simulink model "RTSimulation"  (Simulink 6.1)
settings: Solver=FixedStepDiscrete  StartTime=0.0  StopTime=inf  RelTol=1e-3
PreLoadFcn:
  | initialize
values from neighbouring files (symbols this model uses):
  actParams = [	bulkModulus   * pressCanon    [Copy of initialize.m]    (also in initialize.m = [bulkModulus	* pressCanon,)
  aLpf = [1]    [randth.m]
  bLpf = [1]    [randth.m]
  displFreq = inf    [initialize.m]
  flowCanon = 1.666667e+04    (= 16666.67)    [Copy of initialize.m]    (also in initialize.m)
  forceCanon = 1    [Copy of initialize.m]    (also in initialize.m)
  forceFreq = inf    [initialize.m]
  friction = 5			 				* 0.155000	 				* 0.00444822 				* area1    (= 2.71252900422)    [initialize.m]
  fsamp = 1 / samplePeriod    (= 1024)    [Copy of initialize.m]    (also in initialize.m; rampth.m = 1 / deltaT; randth.m = 1 / deltaT; rspect.m = 1.0 / tsamp)
  gasConstant = 1.8    [Copy of initialize.m]    (also in initialize.m)
  lengthCanon = 1    [Copy of initialize.m]    (also in initialize.m)
  massCanon = 1e-06    [Copy of initialize.m]    (also in initialize.m)
  maxDispl = ( (stroke2 + endLength2) * lengthCanon)'    [Copy of initialize.m]    (also in initialize.m = 576.2)
  maxOilVolume = volume * (1 - (precharge/supplyPress)^(1/gasConstant))    (= 211.391477114)    [Copy of initialize.m]    (also in initialize.m)
  maxVeloc = ( (maxFlow' * flowCanon ./ (area1 * areaCanon)) / velocCanon)'    [Copy of initialize.m]    (also in initialize.m = (maxFlow * flowCanon / (area1 * areaCanon)) / velocCanon; rampth.m = 2 * maxDispl / (nVeloc * deltaT))
  minDispl = (-(stroke1 + endLength1) * lengthCanon)'    [Copy of initialize.m]    (also in initialize.m = -576.2)
  minVeloc = (-(maxFlow' * flowCanon ./ (area2 * areaCanon)) / velocCanon)'    [Copy of initialize.m]    (also in initialize.m = -(maxFlow * flowCanon / (area2 * areaCanon)) / velocCanon)
  nAct = 5    [Copy of initialize.m]    (also in initialize.m = 1)
  nAdcU = 6    [Copy of initialize.m]    (also in initialize.m = 5)
  nDout = 4    [Copy of initialize.m]    (also in initialize.m)
  nDucU = 2    [Copy of initialize.m]    (also in initialize.m)
  nEncU = 3    [Copy of initialize.m]    (also in initialize.m)
  node = completenodestruct(node)    [Copy of initialize.m]    (also in initialize.m)
  precharge = 3000		 				* 6.894757e-03    (= 20.684271)    [Copy of initialize.m]    (also in initialize.m)
  pumpFlow = 1e20    (= 1e+20)    [Copy of initialize.m]    (also in initialize.m)
  returnPress = 3			 				* 0.1    (= 0.3)    [Copy of initialize.m]    (also in initialize.m)
  samplePeriod = controlPeriod/upsampleFactor    (= 0.0009765625)    [Copy of initialize.m]    (also in initialize.m; viewer.m = eval(getHeaderValue(header, 'DELTA_T')))
  springCanon = 1    [Copy of initialize.m]    (also in initialize.m)
  supplyPress = 280		 				* 0.1    (= 28)    [Copy of initialize.m]    (also in initialize.m)
  velocCanon = 1    [Copy of initialize.m]    (also in initialize.m)
  volume = 15.15		 				+ (  45		 				    * 2		 				   + 30		 				    * 6 )	 				* 5    (= 1365.15)    [Copy of initialize.m]    (also in initialize.m; quake.m = volume / 231.0)
  volumeCanon = 1e+06    (= 1000000)    [Copy of initialize.m]    (also in initialize.m)
  yieldDispl = 1.0    (= 1)    [initialize.m]
undefined symbols (not defined in the file or in its folder): DiscIntNeverNeededParam, dpforceFreq, mass, spring, staticForce
libraries: xpclib x6, simulink x1
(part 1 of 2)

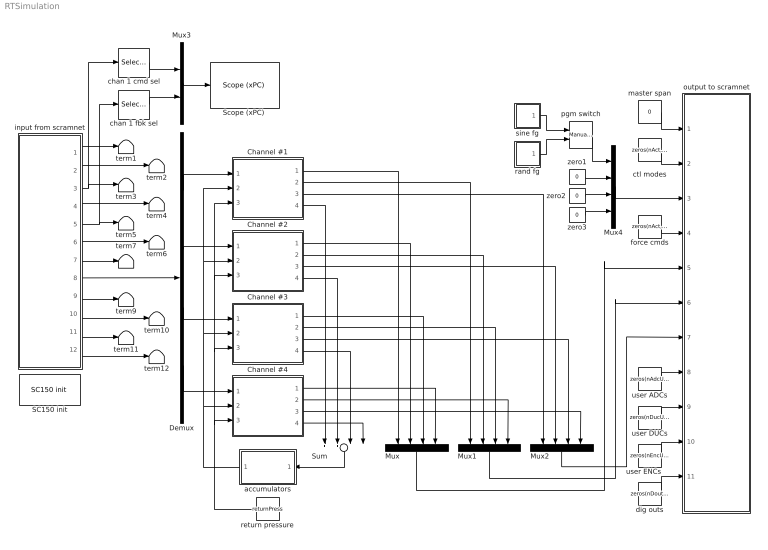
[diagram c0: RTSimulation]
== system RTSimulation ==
  Channel #1 : Subsystem  mask{id=1}
      mask prompts: id "Channel ID"
  Channel #2 : Subsystem  mask{id=2}
      mask prompts: id "Channel ID"
  Channel #3 : Subsystem  mask{id=3}
      mask prompts: id "Channel ID"
  Channel #4 : Subsystem  mask{id=4}
      mask prompts: id "Channel ID"
  Demux : Demux  Outputs=nAct
  Mux : Mux  Orientation=down  Inputs=nAct
  Mux1 : Mux  Orientation=down  Inputs=nAct
  Mux2 : Mux  Orientation=down  Inputs=nAct
  Mux3 : Mux  Inputs=2
  Mux4 : Mux  Inputs=nAct
  SC150 init : xpclib/Shared Memory/Systran/SC150 init   node=node  pci=-1
  "Scope (xPC) " : xpclib/Misc./Scope (xPC)   scopeno=2  scopetype=Target  autostart=on  viewmode=Graphical redraw  formatstr='%15.6f'  grid=on  ylimits=[0,0]  nosamples=1024  noprepostsamples=0  interleave=1  triggermode=FreeRun  triggersignal=1  triggerlevel=0.0  triggerslope=Either  triggerscope=1  triggersample=0  filename=data.dat  mode=Lazy  writesize=512  autorestart=off
  Sum : Sum  Orientation=down  Inputs=++++
  accumulators : Subsystem  Orientation=left
  chan 1 cmd sel : Selector
  chan 1 fbk sel : Selector
  ctl modes : Constant  Value=zeros(nAct, 1)
  dig outs : Constant  Value=zeros(nDout, 1)  OutDataTypeMode=uint32
  force cmds : Constant  Value=zeros(nAct, 1)
  input from scramnet : Subsystem
  master span : Constant  Value=0
  output to scramnet : Subsystem
  pgm switch : simulink/Signal Routing/Manual Switch  sw=1  action=0
  rand fg : Subsystem  mask(Sine Function Generator){ampl=1, bw=10, spanInterval=1, samplePeriod=samplePeriod}
      mask prompts: ampl "RMS amplitude"; bw "Bandwidth (Hz)"; spanInterval "Span interval (sec)"; samplePeriod "Sample period (sec)"
      mask init:
      | gain = ampl*sqrt(3)*sqrt(1/(2*samplePeriod*bw));
  return pressure : Constant  Orientation=left  Value=returnPress
  sine fg : Subsystem  mask(Sine Function Generator){ampl=1, freq=1, spanInterval=1, samplePeriod=samplePeriod}
      mask prompts: ampl "Amplitude"; freq "Frequency (Hz)"; spanInterval "Span interval (sec)"; samplePeriod "Sample period (sec)"
  term{1..7,9..12} (11 alike) : Terminator
  user ADCs : Constant  Value=zeros(nAdcU, 1)
  user DUCs : Constant  Value=zeros(nDucU, 1)
  user ENCs : Constant  Value=zeros(nEncU, 1)
  zero1 : Constant  Value=0
  zero2 : Constant  Value=0
  zero3 : Constant  Value=0
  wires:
  input from scramnet/6(force fbks) -> term6/1
  input from scramnet/10(user ducs) -> term10/1
  input from scramnet/12(dig inps) -> term12/1
  input from scramnet/4(force cmds) -> term4/1
  input from scramnet/5(displ fbks) -> term5/1, chan 1 fbk sel/1
  input from scramnet/7(dpforce fbks) -> term7/1
  input from scramnet/9(user adcs) -> term9/1
  input from scramnet/11(user encs) -> term11/1
  input from scramnet/1(master span) -> term1/1
  input from scramnet/2(ctl modes) -> term2/1
  input from scramnet/3(displ cmds) -> term3/1, chan 1 cmd sel/1
  master span/1 -> output to scramnet/1(master span)
  ctl modes/1 -> output to scramnet/2(ctl modes)
  force cmds/1 -> output to scramnet/4(force cmds)
  user ADCs/1 -> output to scramnet/8(user adcs)
  user DUCs/1 -> output to scramnet/9(user ducs)
  user ENCs/1 -> output to scramnet/10(user encs)
  dig outs/1 -> output to scramnet/11(dig outs)
  Channel #1/4(flow) -> Sum/1
  Channel #2/4(flow) -> Sum/2
  Channel #3/4(flow) -> Sum/3
  Sum/1 -> accumulators/1(flow)
  Channel #4/4(flow) -> Sum/4
  Channel #1/1(displ) -> Mux/1
  Channel #2/1(displ) -> Mux/2
  Channel #3/1(displ) -> Mux/3
  Channel #4/1(displ) -> Mux/4
  Channel #1/2(force) -> Mux1/1
  Channel #2/2(force) -> Mux1/2
  Channel #3/2(force) -> Mux1/3
  Channel #4/2(force) -> Mux1/4
  Channel #1/3(dpforce) -> Mux2/1
  Channel #2/3(dpforce) -> Mux2/2
  Channel #3/3(dpforce) -> Mux2/3
  Channel #4/3(dpforce) -> Mux2/4
  Mux/1 -> output to scramnet/5(displ fbks)
  Mux1/1 -> output to scramnet/6(force fbks)
  Mux2/1 -> output to scramnet/7(dpforce fbks)
  Demux/1 -> Channel #1/1(valve cmd)
  Demux/2 -> Channel #2/1(valve cmd)
  Demux/3 -> Channel #3/1(valve cmd)
  Demux/4 -> Channel #4/1(valve cmd)
  accumulators/1(press) -> Channel #3/2(spl press), Channel #2/2(spl press), Channel #1/2(spl press), Channel #4/2(spl press)
  return pressure/1 -> Channel #3/3(rtn press), Channel #2/3(rtn press), Channel #1/3(rtn press), Channel #4/3(rtn press)
  input from scramnet/8(valve cmds) -> Demux/1
  sine fg/1(out) -> pgm switch/1
  rand fg/1(out) -> pgm switch/2
  chan 1 cmd sel/1 -> Mux3/1
  chan 1 fbk sel/1 -> Mux3/2
  Mux3/1 -> "Scope (xPC) "/1
  zero1/1 -> Mux4/2
  zero2/1 -> Mux4/3
  zero3/1 -> Mux4/4
  Mux4/1 -> output to scramnet/3(displ cmds)
  pgm switch/1 -> Mux4/1

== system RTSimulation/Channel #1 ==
  valve cmd : Inport  Port=1  LatchInput=off
  spl press : Inport  Port=2  LatchInput=off
  rtn press : Inport  Port=3  LatchInput=off
  actuator/valve  model : Subsystem
  displ cond filter : Subsystem  mask{freq3dB=displFreq(id), fsamp=fsamp}
      mask prompts: freq3dB "3 dB cutoff frequency (inf, 500, 300, 100, 50 Hz)"; fsamp "Sampling frequency (Hz)"
      mask init:
      | if isempty(freq3dB)
      | 	freq3dB = fsamp;
      | elseif freq3dB == 500
      | 	freq3dB = 485;
      | elseif freq3dB == 300
      | 	freq3dB = 204.9;
      | elseif freq3dB == 100
      | 	freq3dB = 56.5;
      | elseif freq3dB == 50
      | 	freq3dB = 27.8;
      | else
      | 	freq3dB = fsamp;
      | end
      | if freq3dB > fsamp/2
      | 	a = [1];
      | 	b = [1];
      | else
      | 	[b, a] = ellip(4, 0.001, 60.0, 2*freq3dB/fsamp);
      | end
  dpforce cond filter : Subsystem  mask{freq3dB=dpforceFreq(id), fsamp=fsamp}
      mask prompts: freq3dB "3 dB cutoff frequency (inf, 500, 300, 100, 50 Hz)"; fsamp "Sampling frequency (Hz)"
      mask init:
      | if isempty(freq3dB)
      | 	freq3dB = fsamp;
      | elseif freq3dB == 500
      | 	freq3dB = 485;
      | elseif freq3dB == 300
      | 	freq3dB = 204.9;
      | elseif freq3dB == 100
      | 	freq3dB = 56.5;
      | elseif freq3dB == 50
      | 	freq3dB = 27.8;
      | else
      | 	freq3dB = fsamp;
      | end
      | if freq3dB > fsamp/2
      | 	a = [1];
      | 	b = [1];
      | else
      | 	[b, a] = ellip(4, 0.001, 60.0, 2*freq3dB/fsamp);
      | end
  force cond filter : Subsystem  mask{freq3dB=forceFreq((id)), fsamp=fsamp}
      mask prompts: freq3dB "3 dB cutoff frequency (inf, 500, 300, 100, 50 Hz)"; fsamp "Sampling frequency (Hz)"
      mask init:
      | if isempty(freq3dB)
      | 	freq3dB = fsamp;
      | elseif freq3dB == 500
      | 	freq3dB = 485;
      | elseif freq3dB == 300
      | 	freq3dB = 204.9;
      | elseif freq3dB == 100
      | 	freq3dB = 56.5;
      | elseif freq3dB == 50
      | 	freq3dB = 27.8;
      | else
      | 	freq3dB = fsamp;
      | end
      | if freq3dB > fsamp/2
      | 	a = [1];
      | 	b = [1];
      | else
      | 	[b, a] = ellip(4, 0.001, 60.0, 2*freq3dB/fsamp);
      | end
  payload : Subsystem
  displ : Outport
  force : Outport  Port=2
  dpforce : Outport  Port=3
  flow : Outport  Port=4
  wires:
  dpforce cond filter/1(out) -> dpforce/1
  force cond filter/1(out) -> force/1
  displ cond filter/1(out) -> displ/1
  actuator/valve  model/1(force) -> payload/1(force), dpforce cond filter/1(inp), force cond filter/1(inp)
  actuator/valve  model/2(flow) -> flow/1
  spl press/1 -> actuator/valve  model/4(spl press)
  rtn press/1 -> actuator/valve  model/5(rtn press)
  valve cmd/1 -> actuator/valve  model/1(cmd)
  payload/1(displ) -> displ cond filter/1(inp), actuator/valve  model/2(displ)
  payload/2(veloc) -> actuator/valve  model/3(veloc)

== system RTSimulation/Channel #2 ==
  valve cmd : Inport  Port=1  LatchInput=off
  spl press : Inport  Port=2  LatchInput=off
  rtn press : Inport  Port=3  LatchInput=off
  actuator/valve  model : Subsystem
  displ cond filter : Subsystem  mask{freq3dB=displFreq(id), fsamp=fsamp}
      mask prompts: freq3dB "3 dB cutoff frequency (inf, 500, 300, 100, 50 Hz)"; fsamp "Sampling frequency (Hz)"
      mask init:
      | if isempty(freq3dB)
      | 	freq3dB = fsamp;
      | elseif freq3dB == 500
      | 	freq3dB = 485;
      | elseif freq3dB == 300
      | 	freq3dB = 204.9;
      | elseif freq3dB == 100
      | 	freq3dB = 56.5;
      | elseif freq3dB == 50
      | 	freq3dB = 27.8;
      | else
      | 	freq3dB = fsamp;
      | end
      | if freq3dB > fsamp/2
      | 	a = [1];
      | 	b = [1];
      | else
      | 	[b, a] = ellip(4, 0.001, 60.0, 2*freq3dB/fsamp);
      | end
  dpforce cond filter : Subsystem  mask{freq3dB=dpforceFreq(id), fsamp=fsamp}
      mask prompts: freq3dB "3 dB cutoff frequency (inf, 500, 300, 100, 50 Hz)"; fsamp "Sampling frequency (Hz)"
      mask init:
      | if isempty(freq3dB)
      | 	freq3dB = fsamp;
      | elseif freq3dB == 500
      | 	freq3dB = 485;
      | elseif freq3dB == 300
      | 	freq3dB = 204.9;
      | elseif freq3dB == 100
      | 	freq3dB = 56.5;
      | elseif freq3dB == 50
      | 	freq3dB = 27.8;
      | else
      | 	freq3dB = fsamp;
      | end
      | if freq3dB > fsamp/2
      | 	a = [1];
      | 	b = [1];
      | else
      | 	[b, a] = ellip(4, 0.001, 60.0, 2*freq3dB/fsamp);
      | end
  force cond filter : Subsystem  mask{freq3dB=forceFreq((id)), fsamp=fsamp}
      mask prompts: freq3dB "3 dB cutoff frequency (inf, 500, 300, 100, 50 Hz)"; fsamp "Sampling frequency (Hz)"
      mask init:
      | if isempty(freq3dB)
      | 	freq3dB = fsamp;
      | elseif freq3dB == 500
      | 	freq3dB = 485;
      | elseif freq3dB == 300
      | 	freq3dB = 204.9;
      | elseif freq3dB == 100
      | 	freq3dB = 56.5;
      | elseif freq3dB == 50
      | 	freq3dB = 27.8;
      | else
      | 	freq3dB = fsamp;
      | end
      | if freq3dB > fsamp/2
      | 	a = [1];
      | 	b = [1];
      | else
      | 	[b, a] = ellip(4, 0.001, 60.0, 2*freq3dB/fsamp);
      | end
  payload : Subsystem
  displ : Outport
  force : Outport  Port=2
  dpforce : Outport  Port=3
  flow : Outport  Port=4
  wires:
  payload/2(veloc) -> actuator/valve  model/3(veloc)
  payload/1(displ) -> actuator/valve  model/2(displ), displ cond filter/1(inp)
  valve cmd/1 -> actuator/valve  model/1(cmd)
  rtn press/1 -> actuator/valve  model/5(rtn press)
  spl press/1 -> actuator/valve  model/4(spl press)
  actuator/valve  model/2(flow) -> flow/1
  actuator/valve  model/1(force) -> force cond filter/1(inp), dpforce cond filter/1(inp), payload/1(force)
  displ cond filter/1(out) -> displ/1
  force cond filter/1(out) -> force/1
  dpforce cond filter/1(out) -> dpforce/1

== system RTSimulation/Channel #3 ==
  valve cmd : Inport  Port=1  LatchInput=off
  spl press : Inport  Port=2  LatchInput=off
  rtn press : Inport  Port=3  LatchInput=off
  actuator/valve  model : Subsystem
  displ cond filter : Subsystem  mask{freq3dB=displFreq(id), fsamp=fsamp}
      mask prompts: freq3dB "3 dB cutoff frequency (inf, 500, 300, 100, 50 Hz)"; fsamp "Sampling frequency (Hz)"
      mask init:
      | if isempty(freq3dB)
      | 	freq3dB = fsamp;
      | elseif freq3dB == 500
      | 	freq3dB = 485;
      | elseif freq3dB == 300
      | 	freq3dB = 204.9;
      | elseif freq3dB == 100
      | 	freq3dB = 56.5;
      | elseif freq3dB == 50
      | 	freq3dB = 27.8;
      | else
      | 	freq3dB = fsamp;
      | end
      | if freq3dB > fsamp/2
      | 	a = [1];
      | 	b = [1];
      | else
      | 	[b, a] = ellip(4, 0.001, 60.0, 2*freq3dB/fsamp);
      | end
  dpforce cond filter : Subsystem  mask{freq3dB=dpforceFreq(id), fsamp=fsamp}
      mask prompts: freq3dB "3 dB cutoff frequency (inf, 500, 300, 100, 50 Hz)"; fsamp "Sampling frequency (Hz)"
      mask init:
      | if isempty(freq3dB)
      | 	freq3dB = fsamp;
      | elseif freq3dB == 500
      | 	freq3dB = 485;
      | elseif freq3dB == 300
      | 	freq3dB = 204.9;
      | elseif freq3dB == 100
      | 	freq3dB = 56.5;
      | elseif freq3dB == 50
      | 	freq3dB = 27.8;
      | else
      | 	freq3dB = fsamp;
      | end
      | if freq3dB > fsamp/2
      | 	a = [1];
      | 	b = [1];
      | else
      | 	[b, a] = ellip(4, 0.001, 60.0, 2*freq3dB/fsamp);
      | end
  force cond filter : Subsystem  mask{freq3dB=forceFreq((id)), fsamp=fsamp}
      mask prompts: freq3dB "3 dB cutoff frequency (inf, 500, 300, 100, 50 Hz)"; fsamp "Sampling frequency (Hz)"
      mask init:
      | if isempty(freq3dB)
      | 	freq3dB = fsamp;
      | elseif freq3dB == 500
      | 	freq3dB = 485;
      | elseif freq3dB == 300
      | 	freq3dB = 204.9;
      | elseif freq3dB == 100
      | 	freq3dB = 56.5;
      | elseif freq3dB == 50
      | 	freq3dB = 27.8;
      | else
      | 	freq3dB = fsamp;
      | end
      | if freq3dB > fsamp/2
      | 	a = [1];
      | 	b = [1];
      | else
      | 	[b, a] = ellip(4, 0.001, 60.0, 2*freq3dB/fsamp);
      | end
  payload : Subsystem
  displ : Outport
  force : Outport  Port=2
  dpforce : Outport  Port=3
  flow : Outport  Port=4
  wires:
  dpforce cond filter/1(out) -> dpforce/1
  force cond filter/1(out) -> force/1
  displ cond filter/1(out) -> displ/1
  actuator/valve  model/1(force) -> payload/1(force), dpforce cond filter/1(inp), force cond filter/1(inp)
  actuator/valve  model/2(flow) -> flow/1
  spl press/1 -> actuator/valve  model/4(spl press)
  rtn press/1 -> actuator/valve  model/5(rtn press)
  valve cmd/1 -> actuator/valve  model/1(cmd)
  payload/1(displ) -> displ cond filter/1(inp), actuator/valve  model/2(displ)
  payload/2(veloc) -> actuator/valve  model/3(veloc)

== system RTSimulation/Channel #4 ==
  valve cmd : Inport  Port=1  LatchInput=off
  spl press : Inport  Port=2  LatchInput=off
  rtn press : Inport  Port=3  LatchInput=off
  actuator/valve  model : Subsystem
  displ cond filter : Subsystem  mask{freq3dB=displFreq(id), fsamp=fsamp}
      mask prompts: freq3dB "3 dB cutoff frequency (inf, 500, 300, 100, 50 Hz)"; fsamp "Sampling frequency (Hz)"
      mask init:
      | if isempty(freq3dB)
      | 	freq3dB = fsamp;
      | elseif freq3dB == 500
      | 	freq3dB = 485;
      | elseif freq3dB == 300
      | 	freq3dB = 204.9;
      | elseif freq3dB == 100
      | 	freq3dB = 56.5;
      | elseif freq3dB == 50
      | 	freq3dB = 27.8;
      | else
      | 	freq3dB = fsamp;
      | end
      | if freq3dB > fsamp/2
      | 	a = [1];
      | 	b = [1];
      | else
      | 	[b, a] = ellip(4, 0.001, 60.0, 2*freq3dB/fsamp);
      | end
  dpforce cond filter : Subsystem  mask{freq3dB=dpforceFreq(id), fsamp=fsamp}
      mask prompts: freq3dB "3 dB cutoff frequency (inf, 500, 300, 100, 50 Hz)"; fsamp "Sampling frequency (Hz)"
      mask init:
      | if isempty(freq3dB)
      | 	freq3dB = fsamp;
      | elseif freq3dB == 500
      | 	freq3dB = 485;
      | elseif freq3dB == 300
      | 	freq3dB = 204.9;
      | elseif freq3dB == 100
      | 	freq3dB = 56.5;
      | elseif freq3dB == 50
      | 	freq3dB = 27.8;
      | else
      | 	freq3dB = fsamp;
      | end
      | if freq3dB > fsamp/2
      | 	a = [1];
      | 	b = [1];
      | else
      | 	[b, a] = ellip(4, 0.001, 60.0, 2*freq3dB/fsamp);
      | end
  force cond filter : Subsystem  mask{freq3dB=forceFreq((id)), fsamp=fsamp}
      mask prompts: freq3dB "3 dB cutoff frequency (inf, 500, 300, 100, 50 Hz)"; fsamp "Sampling frequency (Hz)"
      mask init:
      | if isempty(freq3dB)
      | 	freq3dB = fsamp;
      | elseif freq3dB == 500
      | 	freq3dB = 485;
      | elseif freq3dB == 300
      | 	freq3dB = 204.9;
      | elseif freq3dB == 100
      | 	freq3dB = 56.5;
      | elseif freq3dB == 50
      | 	freq3dB = 27.8;
      | else
      | 	freq3dB = fsamp;
      | end
      | if freq3dB > fsamp/2
      | 	a = [1];
      | 	b = [1];
      | else
      | 	[b, a] = ellip(4, 0.001, 60.0, 2*freq3dB/fsamp);
      | end
  payload : Subsystem
  displ : Outport
  force : Outport  Port=2
  dpforce : Outport  Port=3
  flow : Outport  Port=4
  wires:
  payload/2(veloc) -> actuator/valve  model/3(veloc)
  payload/1(displ) -> actuator/valve  model/2(displ), displ cond filter/1(inp)
  valve cmd/1 -> actuator/valve  model/1(cmd)
  rtn press/1 -> actuator/valve  model/5(rtn press)
  spl press/1 -> actuator/valve  model/4(spl press)
  actuator/valve  model/2(flow) -> flow/1
  actuator/valve  model/1(force) -> force cond filter/1(inp), dpforce cond filter/1(inp), payload/1(force)
  displ cond filter/1(out) -> displ/1
  force cond filter/1(out) -> force/1
  dpforce cond filter/1(out) -> dpforce/1

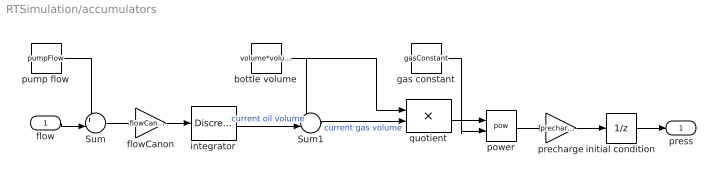
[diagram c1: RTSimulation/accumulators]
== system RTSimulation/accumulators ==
  flow : Inport  Port=1  LatchInput=off
  Sum : Sum  Inputs=+-|
  Sum1 : Sum  Inputs=+-|
  bottle volume : Constant  Value=volume*volumeCanon
  flowCanon : Gain  Gain=flowCanon
  gas constant : Constant  Value=gasConstant
  initial condition : UnitDelay  X0=supplyPress  SampleTime=-1
  integrator : DiscreteIntegrator  InitialCondition=maxOilVolume*volumeCanon  SampleTime=-1  LimitOutput=on  UpperSaturationLimit=maxOilVolume*volumeCanon  LowerSaturationLimit=0  ICPrevOutput=DiscIntNeverNeededParam  ICPrevScaledInput=DiscIntNeverNeededParam
  power : Math  Operator=pow
  precharge : Gain  Gain=precharge
  pump flow : Constant  Value=pumpFlow
  quotient : Product  Inputs=*/
  press : Outport
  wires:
  pump flow/1 -> Sum/1
  Sum/1 -> flowCanon/1
  bottle volume/1 -> Sum1/1, quotient/1
  gas constant/1 -> power/2
  power/1 -> precharge/1
  precharge/1 -> initial condition/1
  Sum1/1 -> quotient/2  "current gas volume"
  quotient/1 -> power/1
  integrator/1 -> Sum1/2  "current oil volume"
  flow/1 -> Sum/2
  flowCanon/1 -> integrator/1
  initial condition/1 -> press/1

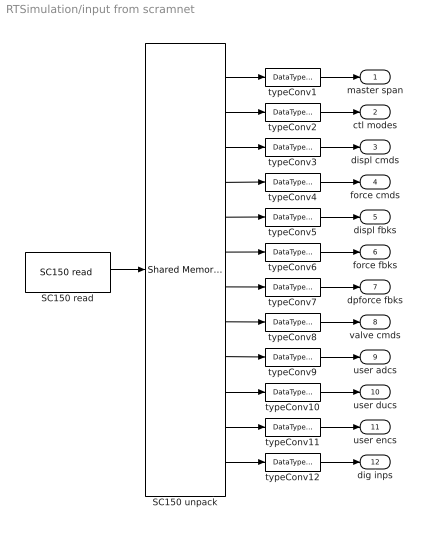
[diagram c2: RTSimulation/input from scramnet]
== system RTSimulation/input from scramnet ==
  SC150 read : xpclib/Shared Memory/Systran/SC150 read   partition=node.Partitions(12:23)  ts=samplePeriod  pci=-1
  SC150 unpack : xpclib/Shared Memory/Shared Memory Unpack   partition=node.Partitions(12:23)
  typeConv{1,3..11} (10 alike) : DataTypeConversion  OutDataTypeMode=double
  typeConv12 : DataTypeConversion  OutDataTypeMode=uint32
  typeConv2 : DataTypeConversion  OutDataTypeMode=uint32
  master span : Outport
  ctl modes : Outport  Port=2
  displ cmds : Outport  Port=3
  force cmds : Outport  Port=4
  displ fbks : Outport  Port=5
  force fbks : Outport  Port=6
  dpforce fbks : Outport  Port=7
  valve cmds : Outport  Port=8
  user adcs : Outport  Port=9
  user ducs : Outport  Port=10
  user encs : Outport  Port=11
  dig inps : Outport  Port=12
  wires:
  typeConv11/1 -> user encs/1
  typeConv10/1 -> user ducs/1
  typeConv12/1 -> dig inps/1
  typeConv9/1 -> user adcs/1
  typeConv8/1 -> valve cmds/1
  typeConv7/1 -> dpforce fbks/1
  typeConv6/1 -> force fbks/1
  typeConv5/1 -> displ fbks/1
  typeConv4/1 -> force cmds/1
  typeConv3/1 -> displ cmds/1
  typeConv1/1 -> master span/1
  SC150 read/1 -> SC150 unpack/1
  typeConv2/1 -> ctl modes/1
  SC150 unpack/1 -> typeConv1/1
  SC150 unpack/2 -> typeConv2/1
  SC150 unpack/3 -> typeConv3/1
  SC150 unpack/4 -> typeConv4/1
  SC150 unpack/5 -> typeConv5/1
  SC150 unpack/6 -> typeConv6/1
  SC150 unpack/7 -> typeConv7/1
  SC150 unpack/8 -> typeConv8/1
  SC150 unpack/9 -> typeConv9/1
  SC150 unpack/10 -> typeConv10/1
  SC150 unpack/11 -> typeConv11/1
  SC150 unpack/12 -> typeConv12/1

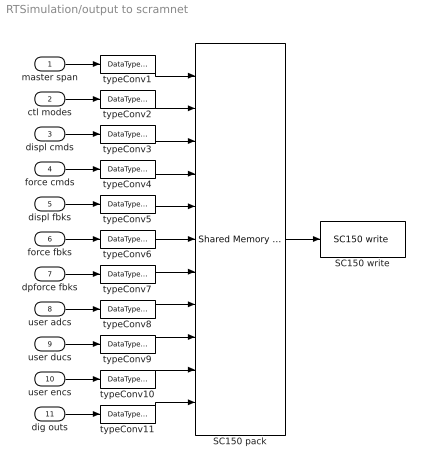
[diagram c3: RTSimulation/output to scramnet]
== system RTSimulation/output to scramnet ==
  master span : Inport  Port=1  LatchInput=off
  ctl modes : Inport  Port=2  LatchInput=off
  displ cmds : Inport  Port=3  LatchInput=off
  force cmds : Inport  Port=4  LatchInput=off
  displ fbks : Inport  Port=5  LatchInput=off
  force fbks : Inport  Port=6  LatchInput=off
  dpforce fbks : Inport  Port=7  LatchInput=off
  user adcs : Inport  Port=8  LatchInput=off
  user ducs : Inport  Port=9  LatchInput=off
  user encs : Inport  Port=10  LatchInput=off
  dig outs : Inport  Port=11  LatchInput=off
  SC150 pack : xpclib/Shared Memory/Shared Memory Pack   partition=node.Partitions(1:11)
  SC150 write : xpclib/Shared Memory/Systran/SC150 write   partition=node.Partitions(1:11)  ts=samplePeriod  pci=-1
  typeConv{1,3..10} (9 alike) : DataTypeConversion  OutDataTypeMode=single
  typeConv11 : DataTypeConversion  OutDataTypeMode=uint32
  typeConv2 : DataTypeConversion  OutDataTypeMode=uint32
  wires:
  typeConv11/1 -> SC150 pack/11
  typeConv10/1 -> SC150 pack/10
  typeConv9/1 -> SC150 pack/9
  typeConv8/1 -> SC150 pack/8
  typeConv7/1 -> SC150 pack/7
  typeConv6/1 -> SC150 pack/6
  typeConv5/1 -> SC150 pack/5
  dig outs/1 -> typeConv11/1
  user encs/1 -> typeConv10/1
  user ducs/1 -> typeConv9/1
  user adcs/1 -> typeConv8/1
  dpforce fbks/1 -> typeConv7/1
  force fbks/1 -> typeConv6/1
  displ fbks/1 -> typeConv5/1
  force cmds/1 -> typeConv4/1
  master span/1 -> typeConv1/1
  SC150 pack/1 -> SC150 write/1
  displ cmds/1 -> typeConv3/1
  ctl modes/1 -> typeConv2/1
  typeConv1/1 -> SC150 pack/1
  typeConv2/1 -> SC150 pack/2
  typeConv3/1 -> SC150 pack/3
  typeConv4/1 -> SC150 pack/4

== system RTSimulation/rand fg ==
  Product : Product
  integrator : DiscreteIntegrator  SampleTime=-1  LimitOutput=on  UpperSaturationLimit=1  LowerSaturationLimit=0  ICPrevOutput=DiscIntNeverNeededParam  ICPrevScaledInput=DiscIntNeverNeededParam
  lowpass : Subsystem  mask{freq=bw, k=gain, samplePeriod=samplePeriod}
      mask prompts: freq "Cutoff frequency (Hz)"; k "Gain"; samplePeriod "Sample period (sec)"
      mask init:
      | damp = sqrt(2);
      | b = [0 0 (2*pi*freq)^2];
      | a = [1 2*(2*pi*freq)*damp (2*pi*freq)^2];
      | [bLpf aLpf] = bilinear(b, a, 1/samplePeriod);
  span rate : Constant  Value=1/spanInterval
  uniform rand : UniformRandomNumber  SampleTime=samplePeriod
  out : Outport
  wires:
  integrator/1 -> Product/2
  span rate/1 -> integrator/1
  Product/1 -> out/1
  uniform rand/1 -> lowpass/1(inp)
  lowpass/1(out) -> Product/1

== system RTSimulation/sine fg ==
  Product : Product
  integrator : DiscreteIntegrator  SampleTime=-1  LimitOutput=on  UpperSaturationLimit=1  LowerSaturationLimit=0  ICPrevOutput=DiscIntNeverNeededParam  ICPrevScaledInput=DiscIntNeverNeededParam
  sine : Sin  Amplitude=ampl  Frequency=2 * pi * freq  SampleTime=samplePeriod
  span rate : Constant  Value=1/spanInterval
  out : Outport
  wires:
  Product/1 -> out/1
  sine/1 -> Product/1
  span rate/1 -> integrator/1
  integrator/1 -> Product/2

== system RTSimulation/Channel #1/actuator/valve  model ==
  note: Parameter vector: 1: oil bulk modulus (force/displ^2) 2: servovalve delay (sec) 3: servovalve overlap 4: rated pressure (force/displ^2) 5: rated flow at rated pressure (displ^3/sec) 6: nominal flow at rated pressure (displ^3/sec) 7: actuator piston area 1 (displ^2) 8: actuator piston area 2 (displ^2) 9: actuator usable stroke 1 (displ) 10: actuator usable stroke 2 (displ) 11: actuator end cushion length 1 (displ) 12: actuator end cushion length 2 (displ) 13: actuator parasitic damping factor 14: cross-chamber leakage factor (flow/press) 15: ratio port openings according to area 16: sample period (sec) Conversion factors used for converting signals from external (user) to internal (canonical) units: 17: displacement 18: velocity 19: force 20: pressure 21: flow
  note: Auxiliary diagnostic output vector: 1: valve opening 2: C1 pressure 3: C2 pressure 4: delta pressure 5: force 6: velocity 7: C1 flow 8: C2 flow 9: total flow 10: kinematic flow 11: compressibility flow 12: leakage flow
  note: Note: "1" and "2" denote actuator cylinders on either side of the actuator piston. With positive valve drive, oil is ported into cylinder 1, resulting in positive displacement.
  cmd : Inport  Port=1  LatchInput=off
  displ : Inport  Port=2  LatchInput=off
  veloc : Inport  Port=3  LatchInput=off
  spl press : Inport  Port=4  LatchInput=off
  rtn press : Inport  Port=5  LatchInput=off
  abs : Abs
  actuator : S-Function  FunctionName=actuator  Parameters=actParams(:,id)
  total flow sel : Selector  Elements=9  InputPortWidth=12
  force : Outport
  flow : Outport  Port=2
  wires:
  abs/1 -> flow/1
  actuator/2 -> total flow sel/1
  total flow sel/1 -> abs/1
  spl press/1 -> actuator/4
  rtn press/1 -> actuator/5
  cmd/1 -> actuator/1
  actuator/1 -> force/1
  displ/1 -> actuator/2
  veloc/1 -> actuator/3

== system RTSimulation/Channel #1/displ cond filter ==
  inp : Inport  Port=1  LatchInput=off
  filter : DiscreteFilter  Numerator=b  Denominator=a  SampleTime=-1
  out : Outport
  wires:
  filter/1 -> out/1
  inp/1 -> filter/1

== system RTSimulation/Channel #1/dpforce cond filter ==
  inp : Inport  Port=1  LatchInput=off
  filter : DiscreteFilter  Numerator=b  Denominator=a  SampleTime=-1
  out : Outport
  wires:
  inp/1 -> filter/1
  filter/1 -> out/1

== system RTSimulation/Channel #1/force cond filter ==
  inp : Inport  Port=1  LatchInput=off
  filter : DiscreteFilter  Numerator=b  Denominator=a  SampleTime=-1
  out : Outport
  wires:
  filter/1 -> out/1
  inp/1 -> filter/1

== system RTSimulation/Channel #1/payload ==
  force : Inport  Port=1  LatchInput=off
  Sum : Sum  Inputs=+---
  displ gen : DiscreteIntegrator  IntegratorMethod=Integration: Backward Euler  SampleTime=-1  LimitOutput=on  UpperSaturationLimit=maxDispl(id)  LowerSaturationLimit=minDispl(id)  ShowSaturationPort=on  ICPrevOutput=DiscIntNeverNeededParam  ICPrevScaledInput=DiscIntNeverNeededParam
  div : Product  Inputs=*/
  friction : Subsystem  Orientation=left  mask{friction=friction(id)*forceCanon, yieldDispl=yieldDispl(id)*lengthCanon, hysteresis=0}
      mask prompts: friction "Sliding friction"; yieldDispl "Equiv. yield displacement (in)"; hysteresis "Hysteresis constant"
  mass : Constant  Value=mass(id)*massCanon
  spring : Gain  Orientation=left  Gain=spring(id)*springCanon
  static force : Constant  Value=staticForce(id)*forceCanon
  unit dly : UnitDelay  Orientation=left  SampleTime=-1
  veloc gen : Subsystem  mask{maxVeloc=maxVeloc(id)*velocCanon, minVeloc=minVeloc(id)*velocCanon, maxDispl=maxDispl(id), minDispl=minDispl(id)}
      mask prompts: maxVeloc "Max velocity"; minVeloc "Min velocity"; maxDispl "Max displacement"; minDispl "Min displacement"
  veloc units : Gain  Gain=1/velocCanon
  displ : Outport
  veloc : Outport  Port=2
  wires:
  spring/1 -> Sum/3  "spring force"
  mass/1 -> div/2
  force/1 -> Sum/1  "total force"
  static force/1 -> Sum/4  "static force"
  Sum/1 -> div/1  "inertial force"
  veloc units/1 -> veloc/1
  unit dly/1 -> spring/1
  friction/1(force) -> Sum/2  "friction force"
  displ gen/2 -> veloc gen/3(reset)
  displ gen/1 -> veloc gen/2(displ), unit dly/1, displ/1
  veloc gen/1(veloc) -> displ gen/1, veloc units/1, friction/1(veloc)
  div/1 -> veloc gen/1(accel)

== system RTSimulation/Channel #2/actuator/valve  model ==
  note: Note: "1" and "2" denote actuator cylinders on either side of the actuator piston. With positive valve drive, oil is ported into cylinder 1, resulting in positive displacement.
  note: Auxiliary diagnostic output vector: 1: valve opening 2: C1 pressure 3: C2 pressure 4: delta pressure 5: force 6: velocity 7: C1 flow 8: C2 flow 9: total flow 10: kinematic flow 11: compressibility flow 12: leakage flow
  note: Parameter vector: 1: oil bulk modulus (force/displ^2) 2: servovalve delay (sec) 3: servovalve overlap 4: rated pressure (force/displ^2) 5: rated flow at rated pressure (displ^3/sec) 6: nominal flow at rated pressure (displ^3/sec) 7: actuator piston area 1 (displ^2) 8: actuator piston area 2 (displ^2) 9: actuator usable stroke 1 (displ) 10: actuator usable stroke 2 (displ) 11: actuator end cushion length 1 (displ) 12: actuator end cushion length 2 (displ) 13: actuator parasitic damping factor 14: cross-chamber leakage factor (flow/press) 15: ratio port openings according to area 16: sample period (sec) Conversion factors used for converting signals from external (user) to internal (canonical) units: 17: displacement 18: velocity 19: force 20: pressure 21: flow
  cmd : Inport  Port=1  LatchInput=off
  displ : Inport  Port=2  LatchInput=off
  veloc : Inport  Port=3  LatchInput=off
  spl press : Inport  Port=4  LatchInput=off
  rtn press : Inport  Port=5  LatchInput=off
  abs : Abs
  actuator : S-Function  FunctionName=actuator  Parameters=actParams(:,id)
  total flow sel : Selector  Elements=9  InputPortWidth=12
  force : Outport
  flow : Outport  Port=2
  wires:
  veloc/1 -> actuator/3
  displ/1 -> actuator/2
  actuator/1 -> force/1
  cmd/1 -> actuator/1
  rtn press/1 -> actuator/5
  spl press/1 -> actuator/4
  total flow sel/1 -> abs/1
  actuator/2 -> total flow sel/1
  abs/1 -> flow/1

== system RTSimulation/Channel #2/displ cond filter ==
  inp : Inport  Port=1  LatchInput=off
  filter : DiscreteFilter  Numerator=b  Denominator=a  SampleTime=-1
  out : Outport
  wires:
  inp/1 -> filter/1
  filter/1 -> out/1

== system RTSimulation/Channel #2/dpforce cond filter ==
  inp : Inport  Port=1  LatchInput=off
  filter : DiscreteFilter  Numerator=b  Denominator=a  SampleTime=-1
  out : Outport
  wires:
  filter/1 -> out/1
  inp/1 -> filter/1

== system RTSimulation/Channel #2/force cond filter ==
  inp : Inport  Port=1  LatchInput=off
  filter : DiscreteFilter  Numerator=b  Denominator=a  SampleTime=-1
  out : Outport
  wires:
  inp/1 -> filter/1
  filter/1 -> out/1

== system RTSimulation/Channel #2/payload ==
  force : Inport  Port=1  LatchInput=off
  Sum : Sum  Inputs=+---
  displ gen : DiscreteIntegrator  IntegratorMethod=Integration: Backward Euler  SampleTime=-1  LimitOutput=on  UpperSaturationLimit=maxDispl(id)  LowerSaturationLimit=minDispl(id)  ShowSaturationPort=on  ICPrevOutput=DiscIntNeverNeededParam  ICPrevScaledInput=DiscIntNeverNeededParam
  div : Product  Inputs=*/
  friction : Subsystem  Orientation=left  mask{friction=friction(id)*forceCanon, yieldDispl=yieldDispl(id)*lengthCanon, hysteresis=0}
      mask prompts: friction "Sliding friction"; yieldDispl "Equiv. yield displacement (in)"; hysteresis "Hysteresis constant"
  mass : Constant  Value=mass(id)*massCanon
  spring : Gain  Orientation=left  Gain=spring(id)*springCanon
  static force : Constant  Value=staticForce(id)*forceCanon
  unit dly : UnitDelay  Orientation=left  SampleTime=-1
  veloc gen : Subsystem  mask{maxVeloc=maxVeloc(id)*velocCanon, minVeloc=minVeloc(id)*velocCanon, maxDispl=maxDispl(id), minDispl=minDispl(id)}
      mask prompts: maxVeloc "Max velocity"; minVeloc "Min velocity"; maxDispl "Max displacement"; minDispl "Min displacement"
  veloc units : Gain  Gain=1/velocCanon
  displ : Outport
  veloc : Outport  Port=2
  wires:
  div/1 -> veloc gen/1(accel)
  veloc gen/1(veloc) -> friction/1(veloc), veloc units/1, displ gen/1
  displ gen/1 -> displ/1, unit dly/1, veloc gen/2(displ)
  displ gen/2 -> veloc gen/3(reset)
  friction/1(force) -> Sum/2  "friction force"
  unit dly/1 -> spring/1
  veloc units/1 -> veloc/1
  Sum/1 -> div/1  "inertial force"
  static force/1 -> Sum/4  "static force"
  force/1 -> Sum/1  "total force"
  mass/1 -> div/2
  spring/1 -> Sum/3  "spring force"

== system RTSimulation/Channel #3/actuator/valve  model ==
  note: Parameter vector: 1: oil bulk modulus (force/displ^2) 2: servovalve delay (sec) 3: servovalve overlap 4: rated pressure (force/displ^2) 5: rated flow at rated pressure (displ^3/sec) 6: nominal flow at rated pressure (displ^3/sec) 7: actuator piston area 1 (displ^2) 8: actuator piston area 2 (displ^2) 9: actuator usable stroke 1 (displ) 10: actuator usable stroke 2 (displ) 11: actuator end cushion length 1 (displ) 12: actuator end cushion length 2 (displ) 13: actuator parasitic damping factor 14: cross-chamber leakage factor (flow/press) 15: ratio port openings according to area 16: sample period (sec) Conversion factors used for converting signals from external (user) to internal (canonical) units: 17: displacement 18: velocity 19: force 20: pressure 21: flow
  note: Auxiliary diagnostic output vector: 1: valve opening 2: C1 pressure 3: C2 pressure 4: delta pressure 5: force 6: velocity 7: C1 flow 8: C2 flow 9: total flow 10: kinematic flow 11: compressibility flow 12: leakage flow
  note: Note: "1" and "2" denote actuator cylinders on either side of the actuator piston. With positive valve drive, oil is ported into cylinder 1, resulting in positive displacement.
  cmd : Inport  Port=1  LatchInput=off
  displ : Inport  Port=2  LatchInput=off
  veloc : Inport  Port=3  LatchInput=off
  spl press : Inport  Port=4  LatchInput=off
  rtn press : Inport  Port=5  LatchInput=off
  abs : Abs
  actuator : S-Function  FunctionName=actuator  Parameters=actParams(:,id)
  total flow sel : Selector  Elements=9  InputPortWidth=12
  force : Outport
  flow : Outport  Port=2
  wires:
  abs/1 -> flow/1
  actuator/2 -> total flow sel/1
  total flow sel/1 -> abs/1
  spl press/1 -> actuator/4
  rtn press/1 -> actuator/5
  cmd/1 -> actuator/1
  actuator/1 -> force/1
  displ/1 -> actuator/2
  veloc/1 -> actuator/3

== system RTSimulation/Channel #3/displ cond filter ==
  inp : Inport  Port=1  LatchInput=off
  filter : DiscreteFilter  Numerator=b  Denominator=a  SampleTime=-1
  out : Outport
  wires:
  filter/1 -> out/1
  inp/1 -> filter/1

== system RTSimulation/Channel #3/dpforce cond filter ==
  inp : Inport  Port=1  LatchInput=off
  filter : DiscreteFilter  Numerator=b  Denominator=a  SampleTime=-1
  out : Outport
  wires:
  inp/1 -> filter/1
  filter/1 -> out/1

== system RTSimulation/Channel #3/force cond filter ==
  inp : Inport  Port=1  LatchInput=off
  filter : DiscreteFilter  Numerator=b  Denominator=a  SampleTime=-1
  out : Outport
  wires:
  filter/1 -> out/1
  inp/1 -> filter/1

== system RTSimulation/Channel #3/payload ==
  force : Inport  Port=1  LatchInput=off
  Sum : Sum  Inputs=+---
  displ gen : DiscreteIntegrator  IntegratorMethod=Integration: Backward Euler  SampleTime=-1  LimitOutput=on  UpperSaturationLimit=maxDispl(id)  LowerSaturationLimit=minDispl(id)  ShowSaturationPort=on  ICPrevOutput=DiscIntNeverNeededParam  ICPrevScaledInput=DiscIntNeverNeededParam
  div : Product  Inputs=*/
  friction : Subsystem  Orientation=left  mask{friction=friction(id)*forceCanon, yieldDispl=yieldDispl(id)*lengthCanon, hysteresis=0}
      mask prompts: friction "Sliding friction"; yieldDispl "Equiv. yield displacement (in)"; hysteresis "Hysteresis constant"
  mass : Constant  Value=mass(id)*massCanon
  spring : Gain  Orientation=left  Gain=spring(id)*springCanon
  static force : Constant  Value=staticForce(id)*forceCanon
  unit dly : UnitDelay  Orientation=left  SampleTime=-1
  veloc gen : Subsystem  mask{maxVeloc=maxVeloc(id)*velocCanon, minVeloc=minVeloc(id)*velocCanon, maxDispl=maxDispl(id), minDispl=minDispl(id)}
      mask prompts: maxVeloc "Max velocity"; minVeloc "Min velocity"; maxDispl "Max displacement"; minDispl "Min displacement"
  veloc units : Gain  Gain=1/velocCanon
  displ : Outport
  veloc : Outport  Port=2
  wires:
  spring/1 -> Sum/3  "spring force"
  mass/1 -> div/2
  force/1 -> Sum/1  "total force"
  static force/1 -> Sum/4  "static force"
  Sum/1 -> div/1  "inertial force"
  veloc units/1 -> veloc/1
  unit dly/1 -> spring/1
  friction/1(force) -> Sum/2  "friction force"
  displ gen/2 -> veloc gen/3(reset)
  displ gen/1 -> veloc gen/2(displ), unit dly/1, displ/1
  veloc gen/1(veloc) -> displ gen/1, veloc units/1, friction/1(veloc)
  div/1 -> veloc gen/1(accel)

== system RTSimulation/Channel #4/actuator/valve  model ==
  note: Note: "1" and "2" denote actuator cylinders on either side of the actuator piston. With positive valve drive, oil is ported into cylinder 1, resulting in positive displacement.
  note: Auxiliary diagnostic output vector: 1: valve opening 2: C1 pressure 3: C2 pressure 4: delta pressure 5: force 6: velocity 7: C1 flow 8: C2 flow 9: total flow 10: kinematic flow 11: compressibility flow 12: leakage flow
  note: Parameter vector: 1: oil bulk modulus (force/displ^2) 2: servovalve delay (sec) 3: servovalve overlap 4: rated pressure (force/displ^2) 5: rated flow at rated pressure (displ^3/sec) 6: nominal flow at rated pressure (displ^3/sec) 7: actuator piston area 1 (displ^2) 8: actuator piston area 2 (displ^2) 9: actuator usable stroke 1 (displ) 10: actuator usable stroke 2 (displ) 11: actuator end cushion length 1 (displ) 12: actuator end cushion length 2 (displ) 13: actuator parasitic damping factor 14: cross-chamber leakage factor (flow/press) 15: ratio port openings according to area 16: sample period (sec) Conversion factors used for converting signals from external (user) to internal (canonical) units: 17: displacement 18: velocity 19: force 20: pressure 21: flow
  cmd : Inport  Port=1  LatchInput=off
  displ : Inport  Port=2  LatchInput=off
  veloc : Inport  Port=3  LatchInput=off
  spl press : Inport  Port=4  LatchInput=off
  rtn press : Inport  Port=5  LatchInput=off
  abs : Abs
  actuator : S-Function  FunctionName=actuator  Parameters=actParams(:,id)
  total flow sel : Selector  Elements=9  InputPortWidth=12
  force : Outport
  flow : Outport  Port=2
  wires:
  veloc/1 -> actuator/3
  displ/1 -> actuator/2
  actuator/1 -> force/1
  cmd/1 -> actuator/1
  rtn press/1 -> actuator/5
  spl press/1 -> actuator/4
  total flow sel/1 -> abs/1
  actuator/2 -> total flow sel/1
  abs/1 -> flow/1

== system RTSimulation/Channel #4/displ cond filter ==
  inp : Inport  Port=1  LatchInput=off
  filter : DiscreteFilter  Numerator=b  Denominator=a  SampleTime=-1
  out : Outport
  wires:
  inp/1 -> filter/1
  filter/1 -> out/1

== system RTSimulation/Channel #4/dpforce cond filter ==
  inp : Inport  Port=1  LatchInput=off
  filter : DiscreteFilter  Numerator=b  Denominator=a  SampleTime=-1
  out : Outport
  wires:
  filter/1 -> out/1
  inp/1 -> filter/1

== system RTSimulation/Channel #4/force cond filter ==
  inp : Inport  Port=1  LatchInput=off
  filter : DiscreteFilter  Numerator=b  Denominator=a  SampleTime=-1
  out : Outport
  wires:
  inp/1 -> filter/1
  filter/1 -> out/1

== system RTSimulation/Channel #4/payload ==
  force : Inport  Port=1  LatchInput=off
  Sum : Sum  Inputs=+---
  displ gen : DiscreteIntegrator  IntegratorMethod=Integration: Backward Euler  SampleTime=-1  LimitOutput=on  UpperSaturationLimit=maxDispl(id)  LowerSaturationLimit=minDispl(id)  ShowSaturationPort=on  ICPrevOutput=DiscIntNeverNeededParam  ICPrevScaledInput=DiscIntNeverNeededParam
  div : Product  Inputs=*/
  friction : Subsystem  Orientation=left  mask{friction=friction(id)*forceCanon, yieldDispl=yieldDispl(id)*lengthCanon, hysteresis=0}
      mask prompts: friction "Sliding friction"; yieldDispl "Equiv. yield displacement (in)"; hysteresis "Hysteresis constant"
  mass : Constant  Value=mass(id)*massCanon
  spring : Gain  Orientation=left  Gain=spring(id)*springCanon
  static force : Constant  Value=staticForce(id)*forceCanon
  unit dly : UnitDelay  Orientation=left  SampleTime=-1
  veloc gen : Subsystem  mask{maxVeloc=maxVeloc(id)*velocCanon, minVeloc=minVeloc(id)*velocCanon, maxDispl=maxDispl(id), minDispl=minDispl(id)}
      mask prompts: maxVeloc "Max velocity"; minVeloc "Min velocity"; maxDispl "Max displacement"; minDispl "Min displacement"
  veloc units : Gain  Gain=1/velocCanon
  displ : Outport
  veloc : Outport  Port=2
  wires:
  div/1 -> veloc gen/1(accel)
  veloc gen/1(veloc) -> friction/1(veloc), veloc units/1, displ gen/1
  displ gen/1 -> displ/1, unit dly/1, veloc gen/2(displ)
  displ gen/2 -> veloc gen/3(reset)
  friction/1(force) -> Sum/2  "friction force"
  unit dly/1 -> spring/1
  veloc units/1 -> veloc/1
  Sum/1 -> div/1  "inertial force"
  static force/1 -> Sum/4  "static force"
  force/1 -> Sum/1  "total force"
  mass/1 -> div/2
  spring/1 -> Sum/3  "spring force"

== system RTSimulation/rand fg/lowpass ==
  inp : Inport  Port=1  LatchInput=off
  gain : Gain  Gain=k
  lowpass1 : DiscreteFilter  Numerator=bLpf  Denominator=aLpf  SampleTime=-1
  lowpass2 : DiscreteFilter  Numerator=bLpf  Denominator=aLpf  SampleTime=-1
  lowpass3 : DiscreteFilter  Numerator=bLpf  Denominator=aLpf  SampleTime=-1
  out : Outport
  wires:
  inp/1 -> lowpass1/1
  gain/1 -> out/1
  lowpass1/1 -> lowpass2/1
  lowpass2/1 -> lowpass3/1
  lowpass3/1 -> gain/1

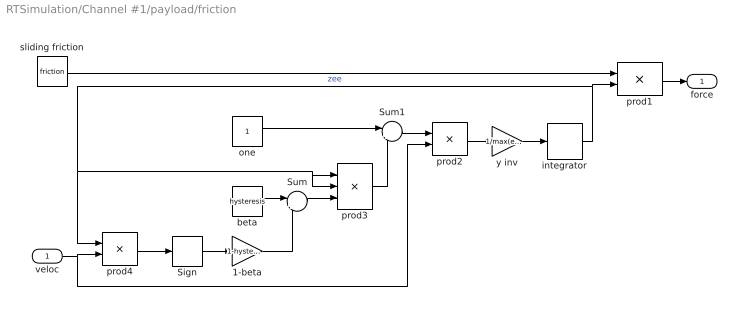
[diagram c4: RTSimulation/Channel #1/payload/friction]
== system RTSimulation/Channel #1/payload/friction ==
  veloc : Inport  Port=1  LatchInput=off
  1-beta : Gain  Gain=1-hysteresis
  Sign : Signum
  Sum : Sum  Inputs=|++
  Sum1 : Sum  Inputs=|+-
  beta : Constant  Value=hysteresis
  integrator : DiscreteIntegrator  SampleTime=-1  LimitOutput=on  UpperSaturationLimit=1  LowerSaturationLimit=-1  ICPrevOutput=DiscIntNeverNeededParam  ICPrevScaledInput=DiscIntNeverNeededParam
  one : Constant
  prod1 : Product
  prod2 : Product
  prod3 : Product  Inputs=3
  prod4 : Product
  sliding friction : Constant  Value=friction
  y inv : Gain  Gain=1/max(eps, yieldDispl)
  force : Outport
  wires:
  integrator/1 -> prod3/2, prod3/1, prod4/1, prod1/2  "zee"
  y inv/1 -> integrator/1
  prod2/1 -> y inv/1
  Sum1/1 -> prod2/1
  prod3/1 -> Sum1/2
  one/1 -> Sum1/1
  Sum/1 -> prod3/3
  beta/1 -> Sum/1
  1-beta/1 -> Sum/2
  Sign/1 -> 1-beta/1
  prod4/1 -> Sign/1
  veloc/1 -> prod2/2, prod4/2
  prod1/1 -> force/1
  sliding friction/1 -> prod1/1

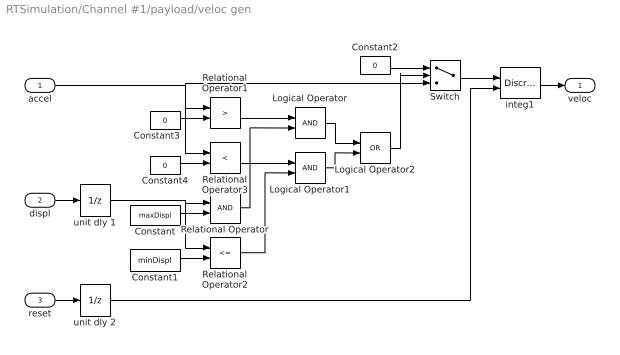
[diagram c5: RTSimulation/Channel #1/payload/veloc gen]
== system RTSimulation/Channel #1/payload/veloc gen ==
  accel : Inport  Port=1  LatchInput=off
  displ : Inport  Port=2  LatchInput=off
  reset : Inport  Port=3  LatchInput=off
  Constant : Constant  Value=maxDispl
  Constant1 : Constant  Value=minDispl
  Constant2 : Constant  Value=0
  Constant3 : Constant  Value=0
  Constant4 : Constant  Value=0
  Logical Operator : Logic
  Logical Operator1 : Logic
  Logical Operator2 : Logic  Operator=OR
  Relational Operator : RelationalOperator
  Relational Operator1 : RelationalOperator  Operator=>
  Relational Operator2 : RelationalOperator  Operator=<=
  Relational Operator3 : RelationalOperator  Operator=<
  Switch : Switch  Threshold=0.5
  integ1 : DiscreteIntegrator  IntegratorMethod=Integration: Backward Euler  ExternalReset=either  SampleTime=-1  LimitOutput=on  UpperSaturationLimit=maxVeloc  LowerSaturationLimit=minVeloc  ICPrevOutput=DiscIntNeverNeededParam  ICPrevScaledInput=DiscIntNeverNeededParam
  unit dly 1 : UnitDelay  SampleTime=-1
  unit dly 2 : UnitDelay  SampleTime=-1
  veloc : Outport
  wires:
  unit dly 1/1 -> Relational Operator2/1, Relational Operator/1
  reset/1 -> unit dly 2/1
  displ/1 -> unit dly 1/1
  Logical Operator1/1 -> Logical Operator2/2
  unit dly 2/1 -> integ1/2
  Switch/1 -> integ1/1
  Logical Operator2/1 -> Switch/2
  Constant2/1 -> Switch/1
  Logical Operator/1 -> Logical Operator2/1
  Relational Operator3/1 -> Logical Operator1/1
  Constant4/1 -> Relational Operator3/2
  Relational Operator1/1 -> Logical Operator/1
  Constant3/1 -> Relational Operator1/2
  accel/1 -> Switch/3, Relational Operator1/1, Relational Operator3/1
  Constant1/1 -> Relational Operator2/2
  Relational Operator2/1 -> Logical Operator1/2
  Relational Operator/1 -> Logical Operator/2
  Constant/1 -> Relational Operator/2
  integ1/1 -> veloc/1

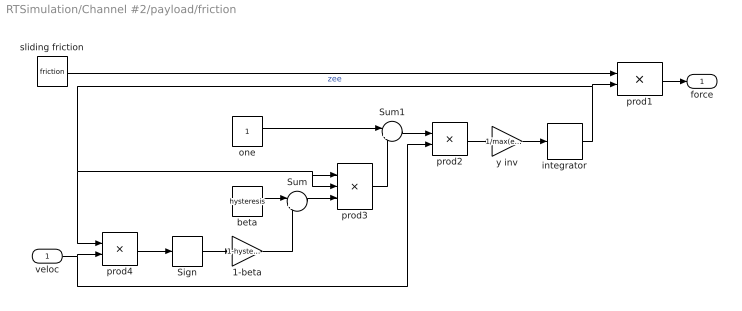
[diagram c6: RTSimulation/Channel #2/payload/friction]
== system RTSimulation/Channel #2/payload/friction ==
  veloc : Inport  Port=1  LatchInput=off
  1-beta : Gain  Gain=1-hysteresis
  Sign : Signum
  Sum : Sum  Inputs=|++
  Sum1 : Sum  Inputs=|+-
  beta : Constant  Value=hysteresis
  integrator : DiscreteIntegrator  SampleTime=-1  LimitOutput=on  UpperSaturationLimit=1  LowerSaturationLimit=-1  ICPrevOutput=DiscIntNeverNeededParam  ICPrevScaledInput=DiscIntNeverNeededParam
  one : Constant
  prod1 : Product
  prod2 : Product
  prod3 : Product  Inputs=3
  prod4 : Product
  sliding friction : Constant  Value=friction
  y inv : Gain  Gain=1/max(eps, yieldDispl)
  force : Outport
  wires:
  sliding friction/1 -> prod1/1
  prod1/1 -> force/1
  veloc/1 -> prod4/2, prod2/2
  prod4/1 -> Sign/1
  Sign/1 -> 1-beta/1
  1-beta/1 -> Sum/2
  beta/1 -> Sum/1
  Sum/1 -> prod3/3
  one/1 -> Sum1/1
  prod3/1 -> Sum1/2
  Sum1/1 -> prod2/1
  prod2/1 -> y inv/1
  y inv/1 -> integrator/1
  integrator/1 -> prod1/2, prod4/1, prod3/1, prod3/2  "zee"

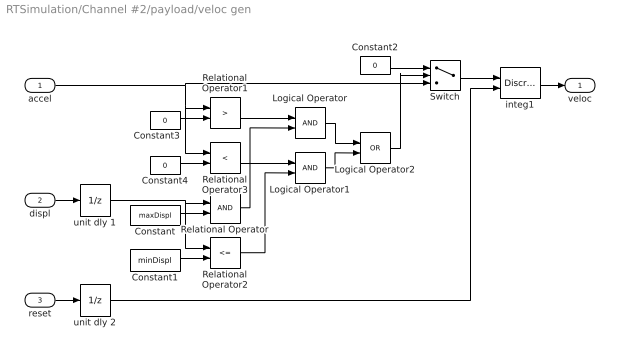
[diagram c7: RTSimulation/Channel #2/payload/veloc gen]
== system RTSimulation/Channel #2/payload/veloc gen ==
  accel : Inport  Port=1  LatchInput=off
  displ : Inport  Port=2  LatchInput=off
  reset : Inport  Port=3  LatchInput=off
  Constant : Constant  Value=maxDispl
  Constant1 : Constant  Value=minDispl
  Constant2 : Constant  Value=0
  Constant3 : Constant  Value=0
  Constant4 : Constant  Value=0
  Logical Operator : Logic
  Logical Operator1 : Logic
  Logical Operator2 : Logic  Operator=OR
  Relational Operator : RelationalOperator
  Relational Operator1 : RelationalOperator  Operator=>
  Relational Operator2 : RelationalOperator  Operator=<=
  Relational Operator3 : RelationalOperator  Operator=<
  Switch : Switch  Threshold=0.5
  integ1 : DiscreteIntegrator  IntegratorMethod=Integration: Backward Euler  ExternalReset=either  SampleTime=-1  LimitOutput=on  UpperSaturationLimit=maxVeloc  LowerSaturationLimit=minVeloc  ICPrevOutput=DiscIntNeverNeededParam  ICPrevScaledInput=DiscIntNeverNeededParam
  unit dly 1 : UnitDelay  SampleTime=-1
  unit dly 2 : UnitDelay  SampleTime=-1
  veloc : Outport
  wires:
  integ1/1 -> veloc/1
  Constant/1 -> Relational Operator/2
  Relational Operator/1 -> Logical Operator/2
  Relational Operator2/1 -> Logical Operator1/2
  Constant1/1 -> Relational Operator2/2
  accel/1 -> Relational Operator3/1, Relational Operator1/1, Switch/3
  Constant3/1 -> Relational Operator1/2
  Relational Operator1/1 -> Logical Operator/1
  Constant4/1 -> Relational Operator3/2
  Relational Operator3/1 -> Logical Operator1/1
  Logical Operator/1 -> Logical Operator2/1
  Constant2/1 -> Switch/1
  Logical Operator2/1 -> Switch/2
  Switch/1 -> integ1/1
  unit dly 2/1 -> integ1/2
  Logical Operator1/1 -> Logical Operator2/2
  displ/1 -> unit dly 1/1
  reset/1 -> unit dly 2/1
  unit dly 1/1 -> Relational Operator/1, Relational Operator2/1
